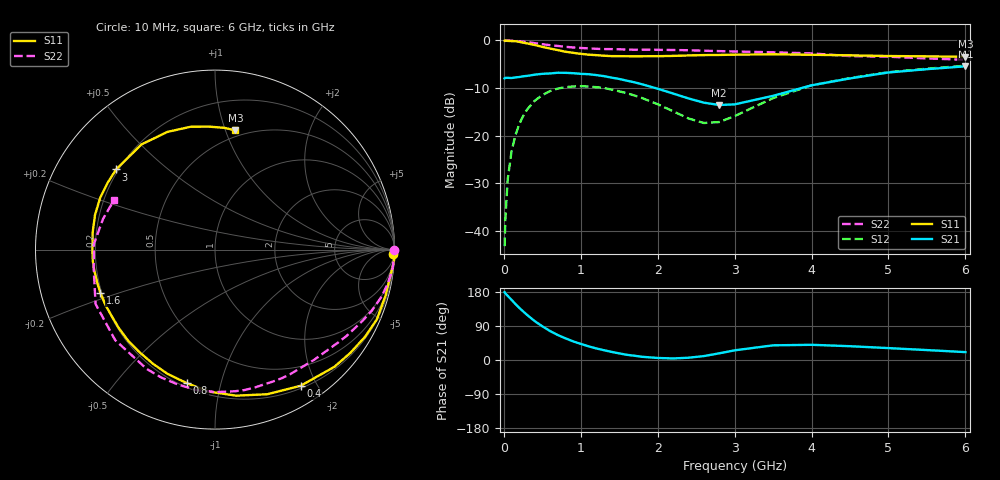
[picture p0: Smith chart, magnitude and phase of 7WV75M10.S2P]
! Infineon Technologies  Discrete & RF Semiconductors
! BFS17W
! Si NPN RF Bipolar Junction Transistor in SOT323
! VCE = 0.75 V  IC = 0.1 mA
! Common Emitter S-Parameters:  August  1999
# GHz  S  MA  R  50
!  f  S11  S21  S12  S22
! GHz  MAG  ANG  MAG  ANG  MAG  ANG  MAG  ANG
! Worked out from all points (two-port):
!   36 points, 10 MHz to 6 GHz, reference 50 ohm
!   highest |S21| = -5.43 dB at 6 GHz (marker M1); lowest = -13.6 dB at 2.8 GHz (marker M2)
!   |S21| within 3 dB of the highest: start of sweep to 1.595 GHz; 4.343 GHz to end of sweep
!   lowest |S11| = -3.4 dB at 6 GHz (marker M3), VSWR 5.14, Z = 22.2 + j54.1 ohm
!   |S11| at or under -10 dB: nowhere
!   |S22| runs from -4.1 to 0.0 dB; largest |S21 - S12| = 0.4
!   S11 on the Smith chart (normalised r, x): 10 MHz: 20, -76; 400 MHz: 0.23, -1.79; 800 MHz: 0.22, -0.79; 1.6 GHz: 0.19, -0.18; 3 GHz: 0.19, +0.34; 6 GHz: 0.44, +1.08
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0.01  0.9935 -1.4  0.4 178.8  0.0069 86.9  0.9999 -0.1
0.02  0.9999 -3.3  0.405 175.8  0.0133 92.3  0.9877 -1.1
0.05  0.9895 -7.6  0.405 169.3  0.0346 85.5  0.998 -2.9
0.1  0.9844 -15.0  0.403 158.8  0.0683 80.0  0.9952 -5.8
0.15  0.982 -23.3  0.409 147.8  0.1008 73.8  0.9879 -8.5
0.2  0.9671 -30.1  0.413 137.7  0.132 69.4  0.9801 -11.3
0.3  0.9322 -44.5  0.424 119.3  0.1871 59.7  0.9607 -16.4
0.4  0.8964 -57.8  0.437 102.8  0.2322 50.5  0.9374 -21.3
0.6  0.8224 -81.7  0.45 76.5  0.2935 35.4  0.8923 -29.6
0.8  0.761 -101.7  0.457 57.2  0.3232 23.4  0.858 -37.3
1.1  0.7091 -126.8  0.442 36.2  0.3284 9.2  0.8259 -48.0
1.3  0.6915 -140.9  0.422 25.9  0.3166 1.8  0.8122 -55.5
1.6  0.6827 -159.2  0.378 13.7  0.2792 -6.7  0.8027 -66.4
2.2  0.6882 172.2  0.277 4.1  0.1804 -7.9  0.7939 -89.6
2.6  0.7018 155.7  0.222 10.3  0.1358 12.6  0.7798 -105.2
2.8  0.7043 148.0  0.21 17.6  0.1389 27.7  0.7731 -112.8
3  0.7092 141.0  0.213 25.5  0.1604 39.8  0.766 -119.8
3.5  0.7151 125.0  0.262 38.7  0.2479 50.1  0.7508 -137.8
4  0.7074 112.0  0.338 40.1  0.3375 46.6  0.7312 -155.5
4.5  0.6978 101.1  0.399 36.4  0.4029 40.2  0.6847 -170.8
5.5  0.6805 85.7  0.499 26.2  0.505 27.9  0.6469 164.7
6  0.6742 80.3  0.535 20.8  0.5429 22.2  0.6269 154.0
